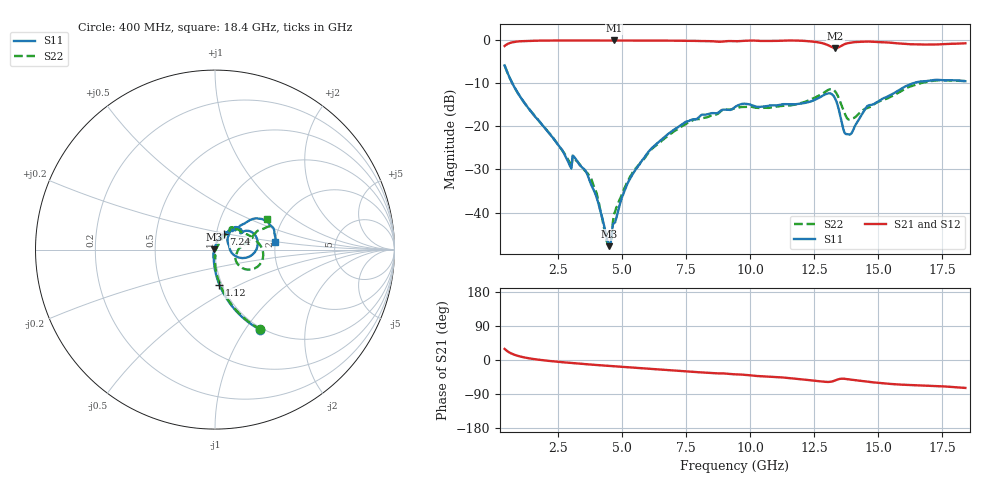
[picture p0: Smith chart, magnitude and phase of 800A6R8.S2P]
!  American Technical Ceramics  Date:  9/12/2007
!  One Norden Lane
!  Huntington Station,  NY.  11746-2102
!  Tel:  (631) 622-4700  Fax:  (631) 622-4748
!  Part Number  800A6R8  Mounting Orientation: Vertical
!  Description: Ultra Low ESR Microwave capacitors
!  Application: Coupling, Bypass, Tuning, DC Block
!  Filters, Matching
# GHZ S DB R 50
! Freq  |S11|  S11 Ph  |S21|  S21 Ph  |S12|  S12 Ph  |S22|  S22 Ph
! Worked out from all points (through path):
!   401 points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, 400 MHz to 18.4 GHz, reference 50 ohm
!   highest |S21| = -0.04 dB at 4.675 GHz (marker M1); lowest = -1.8 dB at 13.31 GHz (marker M2)
!   group delay of S21, straight-line fit = 12.7 ps
!   lowest |S11| = -47.8 dB at 4.495 GHz (marker M3), VSWR 1.01, Z = 49.6 + j0.0796 ohm
!   |S11| at or under -10 dB: 703.1 MHz to 16.35 GHz (15.64 GHz wide, 184 % of centre)
!   |S22| runs from -47.4 to -5.8 dB; largest |S21 - S12| = 0.0019
!   S11 on the Smith chart (normalised r, x): 400 MHz: 0.97, -1.17; 1.12 GHz: 0.97, -0.40; 7.24 GHz: 1.09, +0.19; 18.4 GHz: 1.99, +0.18
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0.4  -5.83 -60.7  -1.33 29.3  -1.33 29.3  -5.82 -60.3
1.12  -14.09 -82.8  -0.19 7.5  -0.18 7.5  -14.08 -81.7
2.92  -28.76 -99.8  -0.05 -7.4  -0.05 -7.4  -28.13 -88.3
3.145  -27.30 -99.3  -0.06 -8.8  -0.06 -8.8  -27.69 -90.2
3.415  -29.48 -100.7  -0.06 -10.3  -0.05 -10.3  -29.44 -90.2
3.865  -34.57 -112.7  -0.06 -12.5  -0.06 -12.6  -33.55 -95.5
4.36  -45.03 -143.9  -0.05 -15.0  -0.05 -15.0  -46.13 -56.7
4.495  -47.82 168.6  -0.05 -15.7  -0.05 -15.7  -47.01 -7.1
4.675  -42.50 100.8  -0.04 -16.5  -0.04 -16.6  -40.41 35.4
5.305  -32.11 80.2  -0.06 -19.6  -0.06 -19.6  -31.63 54.1
6.43  -23.59 68.3  -0.07 -24.8  -0.08 -24.9  -23.90 56.9
7.24  -19.90 60.8  -0.11 -28.8  -0.11 -28.8  -20.27 55.7
9.4  -15.51 45.0  -0.23 -37.8  -0.23 -37.8  -15.77 50.8
12.415  -14.09 31.9  -0.29 -54.0  -0.30 -54.0  -13.58 21.3
13.045  -12.34 14.4  -1.17 -57.9  -1.17 -57.9  -11.52 -0.6
13.315  -13.56 -7.8  -1.81 -53.9  -1.81 -54.0  -11.88 -22.2
13.63  -20.61 -10.1  -1.05 -49.4  -1.05 -49.4  -16.14 -33.2
13.81  -21.82 15.6  -0.67 -50.8  -0.67 -50.9  -18.33 -20.5
14.575  -15.26 46.8  -0.29 -57.1  -0.29 -57.2  -15.73 9.1
15.43  -12.82 41.2  -0.54 -62.9  -0.55 -62.9  -13.27 19.0
16.6  -9.61 27.8  -0.96 -66.9  -0.97 -67.0  -10.07 23.4
18.4  -9.49 6.9  -0.70 -73.7  -0.70 -73.8  -9.47 30.3
